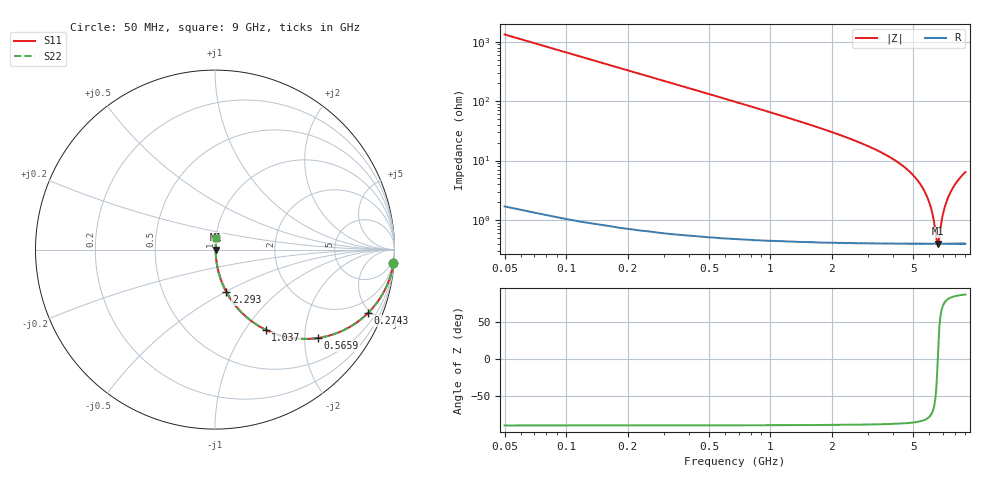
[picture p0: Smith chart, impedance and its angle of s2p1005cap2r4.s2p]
!	AVX	Thin	Film	Operation
!	Date:	March 2012
!	Description: Ultra-Miniature 01005 Size ACCU - P® Thin Film RF / Microwave Capacitor
!	Part Number:  C005YK2R4ABSTR
!	Serial	Measurements
#	MHz	S	db	R	50
!	S11	S21	S12	S22
!	dB	Phase	dB	Phase	dB	Phase	dB	Phase
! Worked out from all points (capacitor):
!   400 points, 50 MHz to 9 GHz, reference 50 ohm
!   read as one part in series: C = 2.4 pF near 94.86 MHz
!   lowest |Z| = 396 mohm at 6.6 GHz (marker M1)
!   series resonance near 6.59 GHz, so ESL is about 240 pH
!   S11 on the Smith chart (normalised r, x): 50 MHz: 1, -27; 274.3 MHz: 1.01, -4.83; 565.9 MHz: 1.01, -2.33; 1.037 GHz: 1.01, -1.25; 2.293 GHz: 1.01, -0.51; 9 GHz: 1.01, +0.13
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50  -0.03 -4.3  -22.48 85.6  -22.48 85.6  -0.03 -4.3
94.862  -0.09 -8.1  -16.98 81.8  -16.98 81.8  -0.09 -8.1
139.724  -0.19 -11.9  -13.71 78.0  -13.71 78.0  -0.19 -11.9
274.311  -0.70 -22.5  -8.35 67.4  -8.35 67.4  -0.70 -22.5
408.897  -1.42 -31.7  -5.59 58.1  -5.59 58.1  -1.42 -31.7
565.915  -2.42 -40.6  -3.73 49.2  -3.73 49.2  -2.42 -40.6
790.226  -3.94 -50.2  -2.29 39.5  -2.29 39.5  -3.94 -50.2
1036.967  -5.55 -57.8  -1.46 31.8  -1.46 31.8  -5.55 -57.8
1552.882  -8.57 -67.5  -0.69 21.9  -0.69 21.9  -8.57 -67.5
2293.108  -12.20 -74.9  -0.30 14.2  -0.30 14.2  -12.20 -74.9
3055.764  -15.53 -79.0  -0.16 9.6  -0.16 9.6  -15.53 -79.0
4536.216  -22.33 -82.7  -0.06 4.4  -0.06 4.4  -22.33 -82.7
5433.459  -28.16 -82.0  -0.04 2.2  -0.04 2.2  -28.16 -82.0
6016.667  -34.56 -76.7  -0.04 1.0  -0.04 1.0  -34.56 -76.7
6240.977  -38.70 -69.5  -0.04 0.6  -0.04 0.6  -38.70 -69.5
6532.581  -47.27 -24.0  -0.03 0.1  -0.03 0.1  -47.27 -24.0
6599.875  -48.03 4.2  -0.03 -0.0  -0.03 -0.0  -48.03 4.2
6869.048  -40.73 64.1  -0.04 -0.5  -0.04 -0.5  -40.73 64.1
7026.065  -37.44 72.1  -0.04 -0.7  -0.04 -0.7  -37.44 72.1
7519.549  -31.44 80.0  -0.04 -1.5  -0.04 -1.5  -31.44 80.0
8147.619  -27.34 82.3  -0.04 -2.5  -0.04 -2.5  -27.34 82.3
9000  -23.95 82.8  -0.05 -3.6  -0.05 -3.6  -23.95 82.8
